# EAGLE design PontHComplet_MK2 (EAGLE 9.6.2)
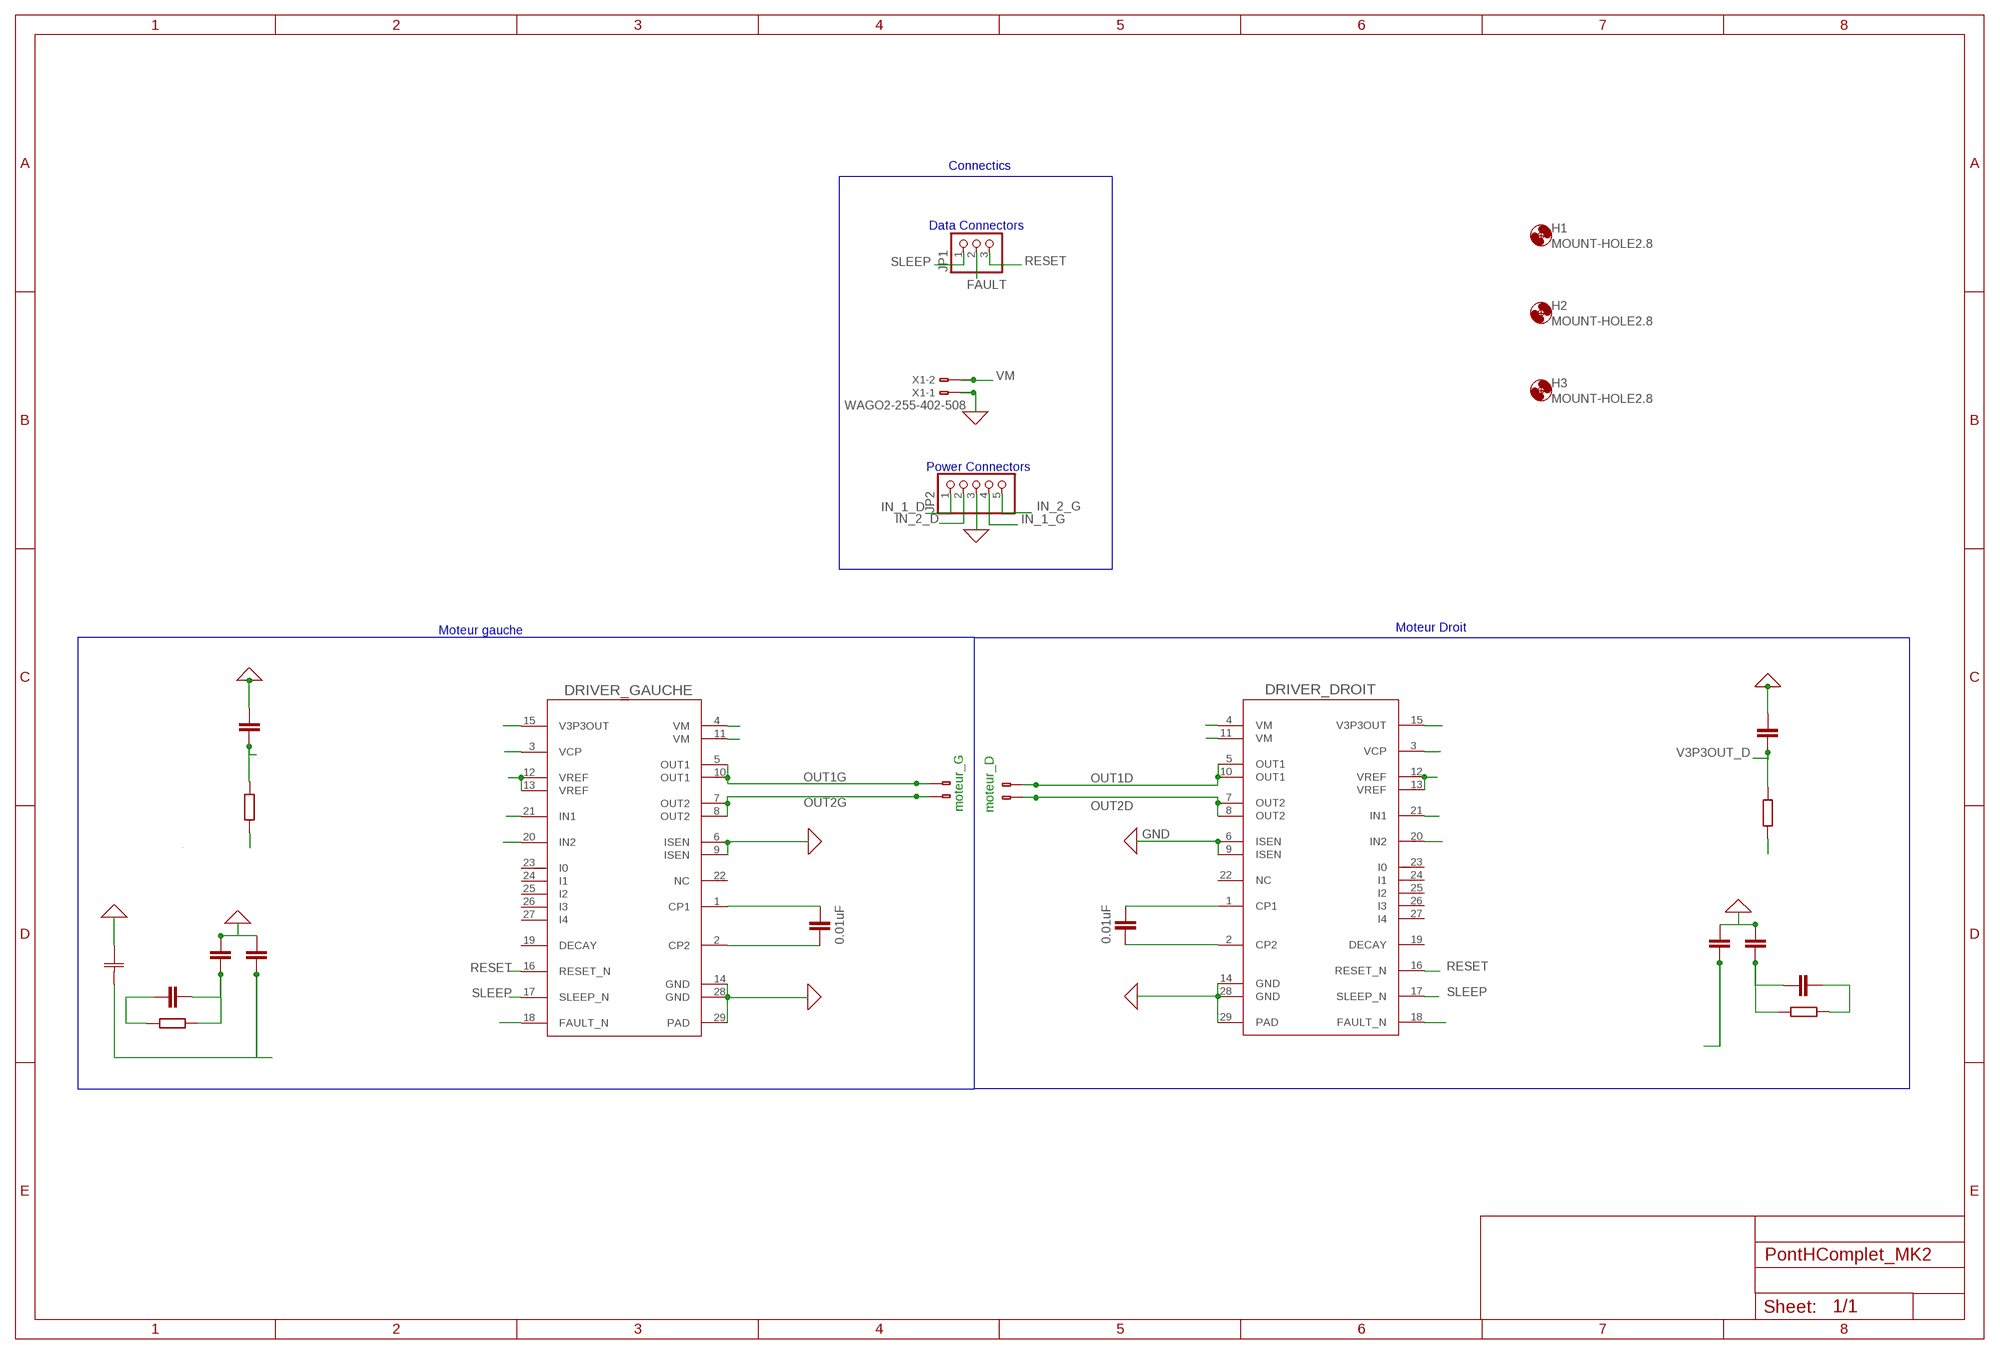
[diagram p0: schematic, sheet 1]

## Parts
D1  0.1uF  C-EUC1206K  [C1206K]
D2  0.1uF  C-EUC1206K  [C1206K]
D3  0.1uF  C-EUC1206K  [C1206K]
D4  1M  R-EU_R1206W  [R1206W]
D5  10K  R-EU_R1206W  [R1206W]
D8  0.47uF  C-EUC1206K  [C1206K]
D10  0.01uF  C-EUC1206K  [C1206K]
DRIVER_DROIT  DRV8842PWPRPWP0028C_M  [PWP0028C_M]
DRIVER_GAUCHE  DRV8842PWPRPWP0028C_M  [PWP0028C_M]
G  220uF  865060557008CAP_60557008_WRE-M  [CAP_60557008_WRE-M]
G1  0.1uF  C-EUC1206K  [C1206K]
G2  0.1uF  C-EUC1206K  [C1206K]
G4  0.1uF  C-EUC1206K  [C1206K]
G5  1M  R-EU_R1206W  [R1206W]
G6  10K  R-EU_R1206W  [R1206W]
G8  0.47uF  C-EUC1206K  [C1206K]
G11  0.01uF  C-EUC1206K  [C1206K]
H1  MOUNT-HOLE2.8  [2,8]
H2  MOUNT-HOLE2.8  [2,8]
H3  MOUNT-HOLE2.8  [2,8]
JP1  PINHD-1X3/90  [1X03/90]
JP2  PINHD-1X5/90  [1X05/90]
MOTEUR_D  WAGO2-255-402-508  [255-402-508]
MOTEUR_G  WAGO2-255-402-508  [255-402-508]
X1  WAGO2-255-402-508  [255-402-508]

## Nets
FAULT: D5.1 DRIVER_DROIT.18(FAULT_N) DRIVER_GAUCHE.18(FAULT_N) G6.1 JP1.2
GND: D1.1 D2.1 D8.1 DRIVER_DROIT.6(ISEN) DRIVER_DROIT.9(ISEN) DRIVER_DROIT.14(GND) DRIVER_DROIT.28(GND) DRIVER_DROIT.29(PAD) DRIVER_GAUCHE.6(ISEN) DRIVER_GAUCHE.9(ISEN) DRIVER_GAUCHE.14(GND) DRIVER_GAUCHE.28(GND) DRIVER_GAUCHE.29(PAD) G1.1 G2.1 G8.1 G.1 JP2.3 X1.A1(-1:A1) X1.B1(-1:B1)
IN_1_D: DRIVER_DROIT.21(IN1) JP2.1
IN_1_G: DRIVER_GAUCHE.21(IN1) JP2.4
IN_2_D: DRIVER_DROIT.20(IN2) JP2.2
IN_2_G: DRIVER_GAUCHE.20(IN2) JP2.5
N$14: D10.2 DRIVER_DROIT.2(CP2)
N$15: D10.1 DRIVER_DROIT.1(CP1)
N$16: DRIVER_GAUCHE.2(CP2) G11.2
N$17: DRIVER_GAUCHE.1(CP1) G11.1
OUT1D [sortie moteur]: DRIVER_DROIT.5(OUT1) DRIVER_DROIT.10(OUT1) MOTEUR_D.A2(-2:A1) MOTEUR_D.B2(-2:B1)
OUT1G [sortie moteur]: DRIVER_GAUCHE.5(OUT1) DRIVER_GAUCHE.10(OUT1) MOTEUR_G.A1(-1:A1) MOTEUR_G.B1(-1:B1)
OUT2D [sortie moteur]: DRIVER_DROIT.7(OUT2) DRIVER_DROIT.8(OUT2) MOTEUR_D.A1(-1:A1) MOTEUR_D.B1(-1:B1)
OUT2G [sortie moteur]: DRIVER_GAUCHE.7(OUT2) DRIVER_GAUCHE.8(OUT2) MOTEUR_G.A2(-2:A1) MOTEUR_G.B2(-2:B1)
RESET: DRIVER_DROIT.16(RESET_N) DRIVER_GAUCHE.16(RESET_N) JP1.3
SLEEP: DRIVER_DROIT.17(SLEEP_N) DRIVER_GAUCHE.17(SLEEP_N) JP1.1
V3P3OUT_D: D5.2 D8.2 DRIVER_DROIT.12(VREF) DRIVER_DROIT.13(VREF) DRIVER_DROIT.15(V3P3OUT)
V3P3OUT_G: DRIVER_GAUCHE.12(VREF) DRIVER_GAUCHE.13(VREF) DRIVER_GAUCHE.15(V3P3OUT) G6.2 G8.2
VCP_D: D3.1 D4.1 DRIVER_DROIT.3(VCP)
VCP_G: DRIVER_GAUCHE.3(VCP) G4.1 G5.1
VM [sortie moteur]: D1.2 D2.2 D3.2 D4.2 DRIVER_DROIT.4(VM) DRIVER_DROIT.11(VM) DRIVER_GAUCHE.4(VM) DRIVER_GAUCHE.11(VM) G1.2 G2.2 G4.2 G5.2 G.2 X1.A2(-2:A1) X1.B2(-2:B1)
Unconnected: DRIVER_DROIT.19(DECAY) DRIVER_DROIT.22(NC) DRIVER_DROIT.23(I0) DRIVER_DROIT.24(I1) DRIVER_DROIT.25(I2) DRIVER_DROIT.26(I3) DRIVER_DROIT.27(I4) DRIVER_GAUCHE.19(DECAY) DRIVER_GAUCHE.22(NC) DRIVER_GAUCHE.23(I0) DRIVER_GAUCHE.24(I1) DRIVER_GAUCHE.25(I2) DRIVER_GAUCHE.26(I3) DRIVER_GAUCHE.27(I4)

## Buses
B$1
B$2
B$3
B$4
B$5

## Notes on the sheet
- Connectics
- Data Connectors
- Power Connectors
- Moteur gauche | Moteur Droit
- moteur_G | moteur_D

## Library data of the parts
D1-D3 D8 D10 G1 G2 G4 G8 G11 = rcl:C-EU: CAPACITOR, European symbol; SPICEPREFIX: C
D4 D5 G5 G6 = rcl:R-EU_: RESISTOR, European symbol; SPICEPREFIX: R
DRIVER_DROIT DRIVER_GAUCHE = driveTexas:DRV8842PWPR; COPYRIGHT: Copyright (C) 2022 Ultra Librarian. All rights reserved.; MANUFACTURER_PART_NUMBER: DRV8842PWPR; MFR_NAME: Texas Instruments; REFDES: RefDes; TYPE: TYPE
G = capacitor cms:865060557008; COPYRIGHT: Copyright (C) 2022 Ultra Librarian. All rights reserved.; MANUFACTURER_PART_NUMBER: 865060557008; MFR_NAME: Wurth Electronics
H1-H3 = holes:MOUNT-HOLE: MOUNTING HOLE with drill center marker
JP1 = pinhead:PINHD-1X3: PIN HEADER
JP2 = pinhead:PINHD-1X5: PIN HEADER
MOTEUR_D MOTEUR_G X1 = con-wago:WAGO2-: WAGO Cage Clamp; OC_FARNELL: unknown; OC_NEWARK: unknown

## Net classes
0 default: width 0.4 mm, drill 0.076 mm
1 sortie moteur: width 0.4 mm, drill 0.3 mm, clearance 0.3 mm to class 0

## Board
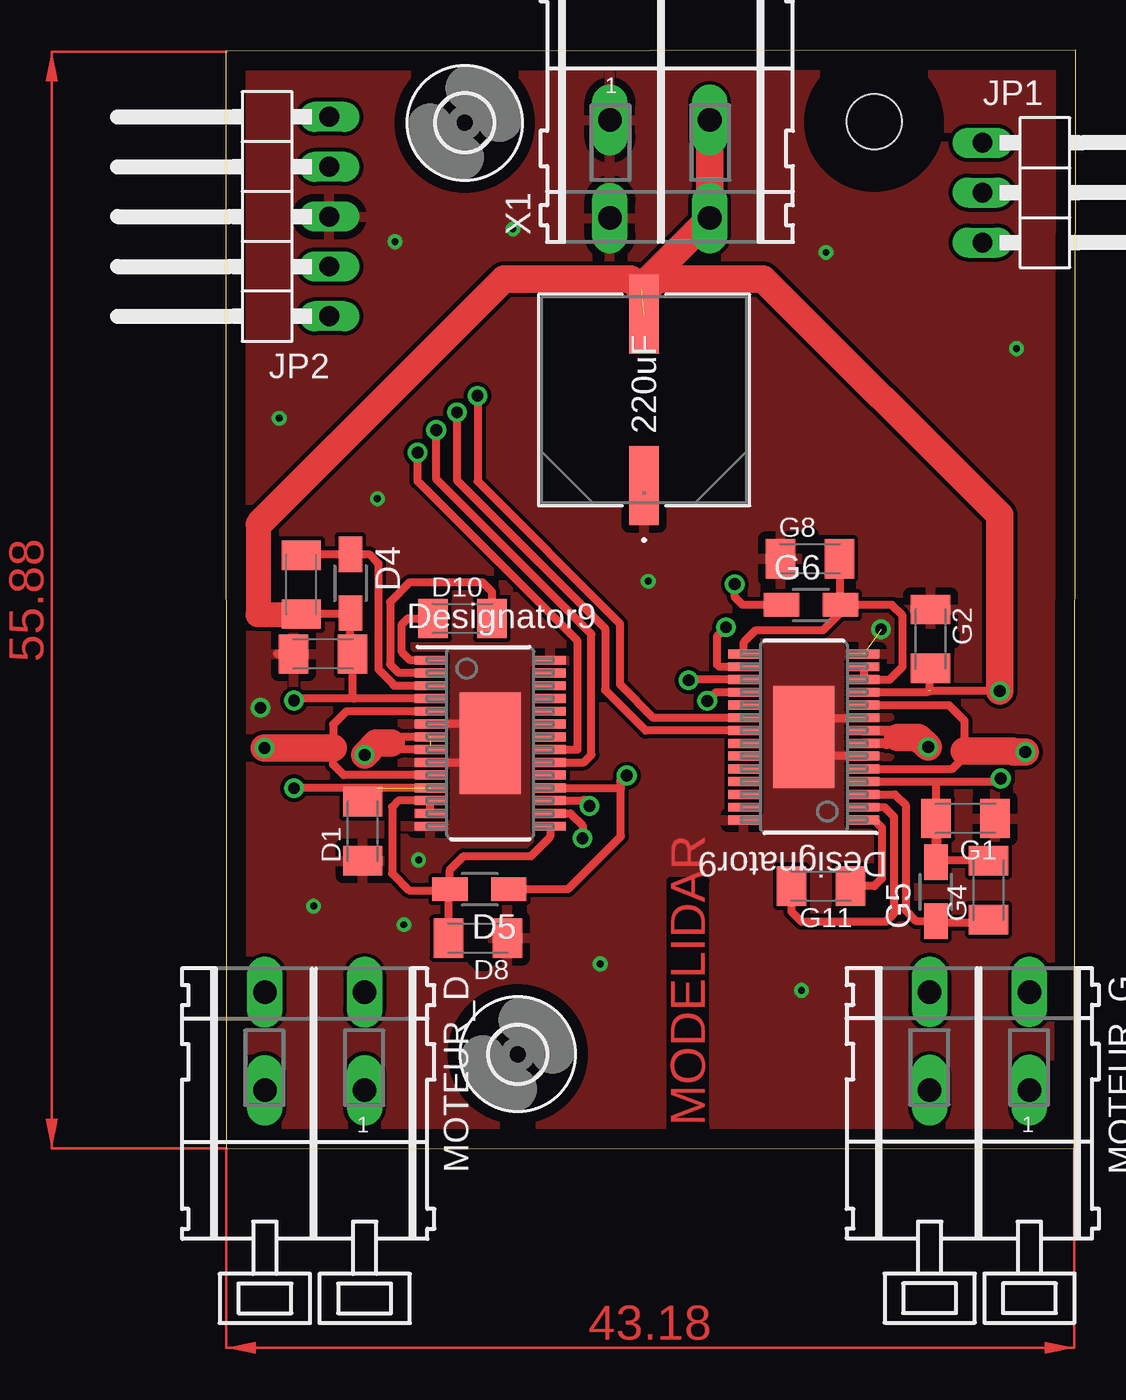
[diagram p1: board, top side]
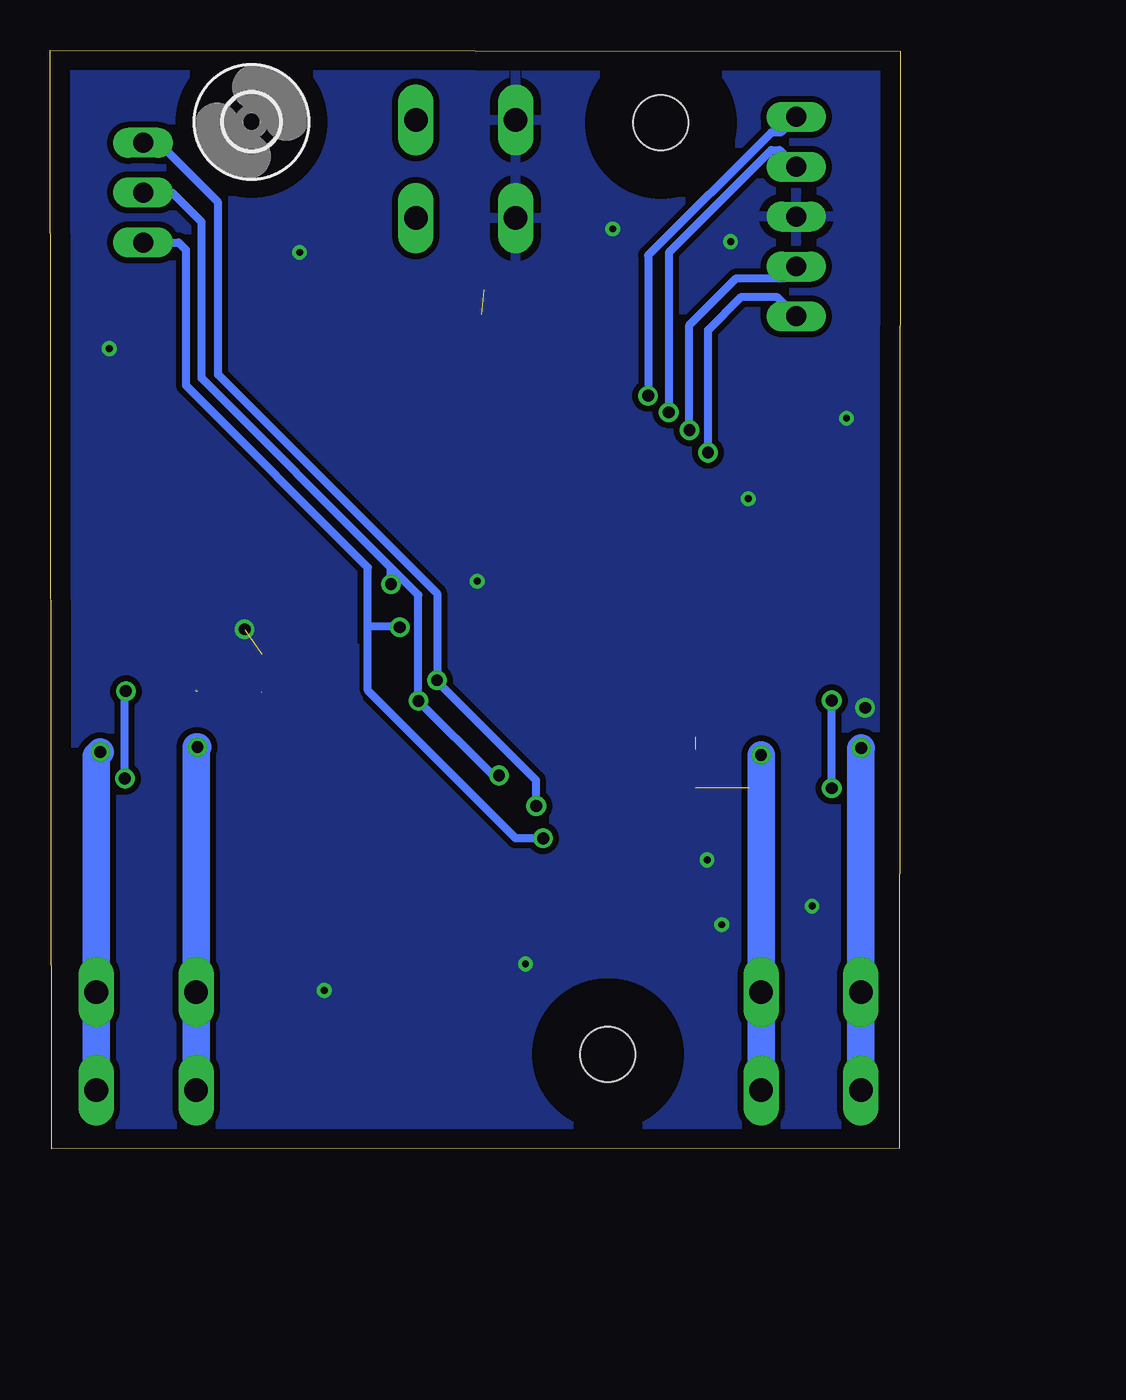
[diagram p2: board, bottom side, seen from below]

Size 43.29 x 55.96 mm. Coordinates in mm from the lower left corner, seen from the top.
Outline: 0.03,0.01 43.21,0 43.29,55.96 0,55.9 0.03,0.01
Copper layers (1*16): Top 0.035mm / dielectric 1.5mm / Bottom 0.035mm
Design rules "design rules *": minimum track width 0.25mm, minimum drill 0.6mm, track to track 0.2mm, track to pad 0.2mm, pad to pad 0.185mm, via to via 0.2mm, smd to smd 0.185mm, copper to edge 1mm, drill to drill 0.4mm, minimum pad ring 0.2mm, minimum via ring 0.2mm, stop-mask expansion 4mil, vias tented up to drill 0mil, thermal gap 0.4mm
tRestrict: area 12.4,9.1 to 13.3,14.3; area 34.8,25.6 to 37.3,26.4; area 29.4,26.7 to 30.1,31.6

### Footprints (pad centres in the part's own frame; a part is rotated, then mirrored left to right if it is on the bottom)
C1206K = smd 1.5 x 2: 1 -1.5,0; 2 1.5,0
R1206W = smd 1.8 x 1.2: 1 -1.499,0; 2 1.499,0
PWP0028C_M = smd 1.6 x 0.45: 1 -3.05,4.225; 2 -3.05,3.575; 3 -3.05,2.925; 4 -3.05,2.275; 5 -3.05,1.625; 6 -3.05,0.975; 7 -3.05,0.325; 8 -3.05,-0.325; 9 -3.05,-0.975; 10 -3.05,-1.625; 11 -3.05,-2.275; 12 -3.05,-2.925; 13 -3.05,-3.575; 14 -3.05,-4.225; 15 3.05,-4.225; 16 3.05,-3.575; 17 3.05,-2.925; 18 3.05,-2.275; 19 3.05,-1.625; 20 3.05,-0.975; 21 3.05,-0.325; 22 3.05,0.325; 23 3.05,0.975; 24 3.05,1.625; 25 3.05,2.275; 26 3.05,2.925; 27 3.05,3.575; 28 3.05,4.225 | smd 3.1 x 5.18: 29 0,0 | smd 0.5 x 0.5: V 0,0
CAP_60557008_WRE-M = smd 4.013 x 1.499: 1 -4.356,0; 2 4.356,0
2,8 = hole 2.8: 0,0
1X03/90 = drill 1.016 long: 1 -2.54,-3.81; 2 0,-3.81; 3 2.54,-3.81
1X05/90 = drill 1.016 long: 1 -5.08,-3.81; 2 -2.54,-3.81; 3 0,-3.81; 4 2.54,-3.81; 5 5.08,-3.81
255-402-508 = drill 1.2 long: A1 -2.54,0; A2 2.54,0; B1 -2.54,-5; B2 2.54,-5

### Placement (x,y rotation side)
D1  6.98,16.17 90 top
D2  4.96,25.2 0 top
D3  3.85,28.74 270 top
D4  6.35,28.79 270 top
D5  12.92,13.21 180 top
D8  12.84,10.73 180 top
D10  12.06,27.01 0 top
DRIVER_DROIT  13.47,20.66 0 top
DRIVER_GAUCHE  29.45,20.97 180 top
G  21.31,38.14 90 top
G1  37.68,16.83 180 top
G2  35.9,25.97 270 top
G4  38.84,13.18 90 top
G5  36.17,13.09 90 top
G6  29.81,27.7 0 top
G8  29.76,30.05 0 top
G11  30.32,13.38 180 top
H1  14.88,4.81 0 top
H2  33.03,52.31 0 bottom
H3  12.18,52.26 0 top
JP1  42.35,48.7 270 top
JP2  1.47,47.49 90 top
MOTEUR_D  4.54,2.97 180 top
MOTEUR_G  38.39,2.98 180 top
X1  22.11,52.41 0 top

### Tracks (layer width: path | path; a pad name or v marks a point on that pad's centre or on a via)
FAULT  (via drill 0.6)
  Top 0.406: 20.13,18.38 20.13,15.91 17.43,13.21 D5.1 | G6.1 26.33,27.7 25.93,28.1 v25.93,28.76 | DRIVER_DROIT.18 20.13,18.38 | 20.13,18.38 20.13,18.71 | DRIVER_GAUCHE.18 24.97,23.25 v24.53,22.81
  Top 0.5: 20.13,18.71 v20.43,19.01
  Bottom 0.406: JP1.2 37.07,48.7 35.57,47.2 35.57,39.25 25.93,29.61 | v25.93,28.76 25.93,29.61 | v20.43,19.01 20.73,19.01 v24.53,22.81 24.53,28.21 25.93,29.61
GND  (via drill 0.35, 0.6)  (1 unrouted)
  Top 0.4: 2.62,25.2 D2.1 | DRIVER_GAUCHE.6 30.42,20 DRIVER_GAUCHE.29 30.42,21.95 DRIVER_GAUCHE.9 | DRIVER_DROIT.9 12.5,19.68 DRIVER_DROIT.29 12.5,21.63 DRIVER_DROIT.6
  Bottom 0.4: 1.78,22.54 v1.78,22.46
  other vias: 33.38,26.46 4.48,12.36 9.08,11.41 9.83,14.71 19.08,9.41 29.33,8.06 40.28,40.76 21.53,28.91 30.58,45.66 8.63,46.21 14.63,46.86 2.73,37.21 7.73,33.11
  pour Top: 0.13,55.86 43.13,55.86 43.13,0.21 0.13,0.21
  pour Bottom (isolate 0.305): 0.13,55.86 43.13,55.86 43.13,0.21 0.13,0.21
  pour Top (no thermals): 11.43,25.31 15.48,25.31 15.48,15.96 11.43,15.96
  pour Top (no thermals): 27.38,25.61 31.43,25.61 31.43,16.31 27.38,16.31
  pour Bottom: 31.48,25.61 31.48,16.36 31.48,16.26 27.43,16.26 27.43,25.61
  pour Bottom: 11.58,25.21 15.38,25.21 15.38,16.06 11.58,16.06 11.58,25.16
IN_1_D  (via drill 0.6)
  Top 0.406: DRIVER_DROIT.21 17.93,20.33 17.93,25.86 9.78,34.01 v9.78,35.46
  Bottom 0.406: JP2.1 6.28,43.41 8.08,43.41 9.78,41.71 v9.78,35.46
IN_1_G  (via drill 0.6)
  Top 0.406: DRIVER_GAUCHE.21 21.39,21.3 19.33,23.36 19.33,26.51 11.78,34.06 v11.78,37.51
  Bottom 0.406: JP2.4 6.13,50.88 6.56,50.88 11.78,45.66 v11.78,37.51
IN_2_D  (via drill 0.6)
  Top 0.406: DRIVER_DROIT.20 18.25,19.68 18.63,20.06 18.63,26.21 10.73,34.11 v10.73,36.61
  Bottom 0.406: v10.73,36.61 10.73,41.96 8.34,44.35 5.88,44.35 JP2.2
IN_2_G  (via drill 0.6)
  Top 0.406: DRIVER_GAUCHE.20 21.79,21.95 20.08,23.66 20.08,26.75 12.83,34 v12.83,38.36
  Bottom 0.406: JP2.5 6.08,51.77 6.57,51.77 12.83,45.51 v12.83,38.36
N$14
  Top 0.406: D10.2 13.56,28.38 13.08,28.86 9.38,28.86 8.38,27.86 8.38,24.67 8.8,24.25 10.4,24.25 DRIVER_DROIT.2
N$15
  Top 0.4: DRIVER_DROIT.1 9.41,24.88 8.98,25.31 8.98,26.71 9.28,27.01 D10.1
N$16
  Top 0.406: DRIVER_GAUCHE.2 33.55,17.4 34.03,16.92 34.03,11.96 33.63,11.56 29.33,11.56 28.82,12.07 G11.2
N$17
  Top 0.406: G11.1 33.04,13.38 33.42,13.76 33.42,16.36 33.03,16.75 DRIVER_GAUCHE.1
OUT1D  (via drill 0.6)
  Top 0.406: DRIVER_DROIT.5 6.15,22.28 5.48,21.61 5.48,20.41 5.48,19.56 6.01,19.03 DRIVER_DROIT.10
  Top 1.4: 5.48,20.41 v1.98,20.41
  Bottom 1.4: MOTEUR_D.A2 MOTEUR_D.B2 1.99,20.39 v1.98,20.41
OUT1G  (via drill 0.6)
  Top 0.406: DRIVER_GAUCHE.5 37.02,19.35 37.63,19.96 | DRIVER_GAUCHE.10 36.84,22.6 37.63,21.81 37.63,20.26
  Top 0.5: 37.63,19.96 37.63,20.26
  Top 1.4: v40.73,20.21 40.11,20.21 40.06,20.26 37.63,20.26
  Bottom 1.4: MOTEUR_G.A1 MOTEUR_G.B1 40.93,20 v40.73,20.21
OUT2D  (via drill 0.6)  (1 unrouted)
  Top 0.406: DRIVER_DROIT.8 8.81,20.33 | 8.48,20.66 8.18,20.96 | 8.43,20.66 8.48,20.66 | DRIVER_DROIT.7 8.9,20.98 8.58,20.66 8.48,20.66
  Top 1.4: v7.08,20.06 7.68,20.66 8.43,20.66
  Bottom 1.4: MOTEUR_D.A1 MOTEUR_D.B1 v7.07,20.06 v7.08,20.06
OUT2G  (via drill 0.6)
  Top 0.5: 33.66,20.65 33.66,20.6 34.23,20.96
  Top 0.508: DRIVER_GAUCHE.8 33.88,21.3 33.88,20.65 33.66,20.65 DRIVER_GAUCHE.7
  Top 1.4: v35.78,20.46 35.28,20.96 34.23,20.96
  Bottom 1.4: v35.78,20.46 35.85,20.46 MOTEUR_G.B2 MOTEUR_G.A2
RESET  (via drill 0.6)
  Top 0.406: DRIVER_DROIT.16 17.56,17.08 18.18,16.46 v18.18,15.81 | DRIVER_GAUCHE.16 25.14,24.55 25.03,24.66 25.03,26.11 v25.48,26.56
  Bottom 0.406: v18.18,15.81 19.58,15.81 27.1,23.33 27.1,26.61 | 27.1,26.61 27.1,29.62 36.38,38.89 36.38,45.8 36.74,46.16 JP1.3 | 25.53,26.61 27.1,26.61
  Bottom 0.5: v25.48,26.56 25.53,26.61
SLEEP  (via drill 0.6)
  Top 0.406: DRIVER_DROIT.17 18.26,17.73 | DRIVER_GAUCHE.17 23.62,23.9
  Top 0.5: 18.26,17.73 v18.53,17.46 | 23.62,23.9 v23.58,23.86
  Bottom 0.406: v23.58,23.86 23.58,28.28 34.73,39.43 34.73,48.21 37.76,51.24 JP1.1 | 23.6,23.84 18.53,18.76 v18.53,17.46
  Bottom 0.5: v23.58,23.86 23.6,23.84
V3P3OUT_D
  Top 0.406: DRIVER_DROIT.13 DRIVER_DROIT.12 8.8,17.73 8.48,17.41 8.48,14.01 9.33,13.16 11.24,13.16 11.28,13.2 | 11.34,13.13 D8.2 | DRIVER_DROIT.15 16.52,15.88 15.55,14.91 12.13,14.91 11.42,14.2 D5.2
  Top 0.5: 11.32,13.11 11.34,13.13 | D5.2 11.34,13.13 | 11.28,13.2 11.34,13.13
V3P3OUT_G
  Top 0.406: DRIVER_GAUCHE.13 DRIVER_GAUCHE.12 33.82,23.9 34.48,24.56 34.48,27.16 33.93,27.7 G6.2 | G6.2 31.31,30 | DRIVER_GAUCHE.15 26.4,25.8 27.01,26.41 30.43,26.41 31.31,27.29 G6.2
  Top 0.5: 31.31,30 G8.2
VCP_D
  Top 0.4: 7.68,29.91 7.77,29.81 7.77,24.42 8.53,23.67 8.53,23.63 8.58,23.58 DRIVER_DROIT.3
  Top 0.406: 3.89,30.29 D4.1 7.3,30.29 7.68,29.91
  Top 0.5: D3.1 3.89,30.29
VCP_G
  Top 0.406: DRIVER_GAUCHE.3 34.09,18.05 34.63,17.51 34.63,12.14 35.18,11.59 G5.1 | 36.18,11.54 38.71,11.54
  Top 0.508: 38.71,11.54 G4.1 | G5.1 36.18,11.54
VM  (via drill 0.6)  (5 unrouted)
  Top 0.4: DRIVER_GAUCHE.4 36.13,18.7 | 36.13,18.7 39.32,18.7 | G1.2 36.18,18.64 36.13,18.7
  Top 0.406: 32.51,23.27 35.76,23.27 35.87,23.37 | 35.87,23.31 35.87,24.43 | v39.42,23.3 35.76,23.3 | DRIVER_DROIT.11 3.5,18.38 | G4.2 36.26,14.68 | 7.69,18.38 D1.2 | D4.2 6.35,25.31 D2.2 6.46,23 6.53,22.93 | 6.3,27.24 D3.2 | DRIVER_DROIT.4 6.53,22.93 | 6.53,22.93 3.58,22.93 v3.48,22.83
  Top 0.5: 35.87,24.43 G2.2 | G5.2 G1.2 36.38,17.02 | 39.32,18.7 v39.48,18.86 | v39.43,23.31 v39.42,23.3 | 3.5,18.38 v3.48,18.36 | 36.26,14.68 G5.2 | 6.46,27.18 D4.2 6.3,27.24
  Top 0.508: 36.3,14.72 G5.2 | 38.76,14.59 G4.2
  Top 1.27: 1.78,31.93 1.65,31.8 1.65,27.21 3.82,27.21 D3.2
  Top 1.4: X1.A2 X1.B2 21.18,43.93 21.18,43.76 | G1.2 36.15,16.8 | G1.2 | 36.2,16.85 G1.2 | 1.78,31.93 14.16,44.31 20.63,44.31 21.28,43.66 21.28,42.52 G.2 21.33,42.52 21.33,43.66 21.98,44.31 27.38,44.31 39.42,32.28 v39.42,23.3
  Bottom 0.406: v39.48,18.86 39.48,23.26 | v3.48,18.36 v3.48,22.83
  Bottom 0.5: 39.48,23.26 v39.43,23.31
(copper drawn outside any net)
  shapes: Top area x2

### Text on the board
Top: MODELIDAR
